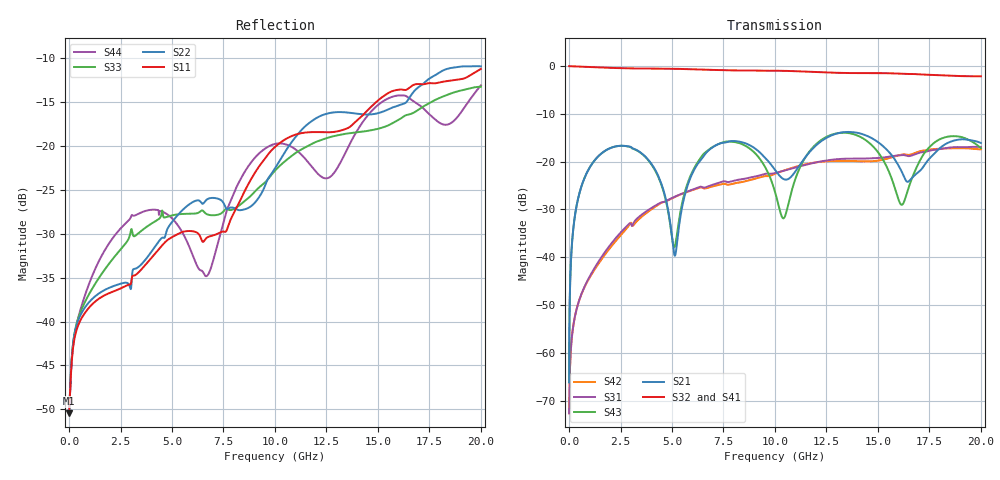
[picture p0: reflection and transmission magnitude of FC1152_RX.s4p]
! Touchstone generated by fitter/viewer
# HZ S  RI R 5.000000e+001
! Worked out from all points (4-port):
!   4999 points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, 4.001 MHz to 20 GHz, reference 50 ohm
!   strongest paths, dB at 4.001 MHz, 5.001 GHz, 10 GHz, 15 GHz, 20 GHz:
!     S32: 0.0, -0.6, -1.0, -1.5, -2.1
!     S41: 0.0, -0.6, -1.0, -1.5, -2.1
!     S21: -66.2, -35.8, -21.7, -15.9, -16.1
!     S43: -66.2, -35.9, -26.3, -18.0, -17.2
!     S31: -72.7, -27.6, -22.4, -19.2, -16.9
!     S42: -72.7, -27.7, -22.5, -19.8, -17.4
!   lowest |S11| = -50.5 dB at 4.001 MHz (marker M1), VSWR 1.01, Z = 50.3 + j0.023 ohm
!   |S11| at or under -10 dB: start of sweep to end of sweep
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4000800  0.00299 0.000229  0.000222 0.000439  -0.000218 -7.98e-05  0.997 -0.00283
         0.000222 0.000439  0.00299 0.000246  0.997 -0.00284  -0.000218 -7.98e-05
         -0.000218 -7.98e-05  0.997 -0.00284  0.00299 0.000247  0.000222 0.000439
         0.997 -0.00283  -0.000218 -7.98e-05  0.000222 0.000439  0.00299 0.000231
3.520704e8  0.00883 -0.000387  0.0085 0.0321  -0.00152 -0.00232  0.9633 -0.2181
            0.0085 0.0321  0.00937 0.000765  0.9631 -0.2188  -0.00155 -0.0023
            -0.00152 -0.00232  0.9631 -0.2188  0.0095 0.00116  0.00839 0.0321
            0.9633 -0.2181  -0.00155 -0.0023  0.00839 0.0321  0.00945 -0.000131
1.580316e9  -0.00362 -0.0133  0.1012 0.0682  -0.00789 -0.00623  0.5511 -0.7904
            0.1012 0.0682  0.00135 -0.0147  0.5487 -0.7922  -0.00764 -0.00568
            -0.00789 -0.00623  0.5487 -0.7922  0.00716 -0.0172  0.1003 0.0698
            0.5511 -0.7904  -0.00764 -0.00568  0.1003 0.0698  0.00664 -0.0227
5.165033e9  0.0263 0.0164  0.0103 0.00275  -0.00386 0.0431  -0.9336 -0.061
            0.0103 0.00275  0.0218 0.0324  -0.9339 -0.051  -0.00411 0.0428
            -0.00386 0.0431  -0.9339 -0.051  -0.0325 0.0244  0.0124 0.00575
            -0.9336 -0.061  -0.00411 0.0428  0.0124 0.00575  -0.0366 0.00499
1.023805e10  0.1027 -0.0176  0.0658 -0.0256  0.00939 -0.0777  0.8682 0.1989
             0.0658 -0.0256  0.083 0.00499  0.8738 0.1807  0.0134 -0.0768
             0.00939 -0.0777  0.8738 0.1807  -0.0748 -0.0194  -0.0197 -0.0238
             0.8682 0.1989  0.0134 -0.0768  -0.0197 -0.0238  -0.0857 -0.0582
1.574715e10  0.1471 -0.1452  0.0385 -0.1041  0.0151 0.1137  -0.8242 -0.1064
             0.0385 -0.1041  0.1195 -0.1161  -0.8338 -0.0805  0.00626 0.1123
             0.0151 0.1137  -0.8338 -0.0805  -0.0963 -0.096  -0.0127 -0.058
             -0.8242 -0.1064  0.00626 0.1123  -0.0127 -0.058  -0.1163 -0.1527
2e10  0.1276 -0.2441  0.0194 -0.1556  0.0546 -0.1318  0.5673 0.5371
      0.0194 -0.1556  0.0934 -0.2691  0.5779 0.5252  0.0527 -0.1239
      0.0546 -0.1318  0.5779 0.5252  0.1818 -0.1203  0.1158 -0.075
      0.5673 0.5371  0.0527 -0.1239  0.1158 -0.075  0.1475 -0.1659
